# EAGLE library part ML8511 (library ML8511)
UV Sensor with Voltage Output Source: Datasheet
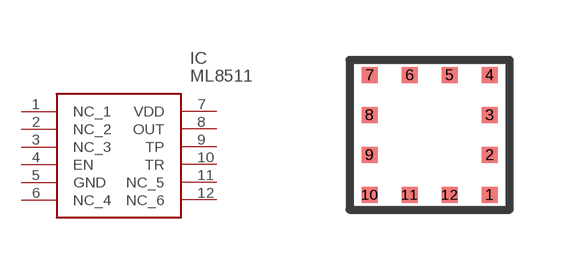
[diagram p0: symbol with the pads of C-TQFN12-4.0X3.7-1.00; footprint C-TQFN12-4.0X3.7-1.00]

Designator prefix IC

## ML8511 (Description: UV Sensor with Voltage Output; Height: mm; Manufacturer_Name: LAPIS SEMICONDUCTOR; Manufacturer_Part_Number: ML8511)  [C-TQFN12-4.0X3.7-1.00]
1  NC_1
2  NC_2
3  NC_3
4  EN
5  GND  pwr
6  NC_4
7  VDD  pwr
8  OUT  out
9  TP
10  TR
11  NC_5
12  NC_6

## Footprint C-TQFN12-4.0X3.7-1.00 (pad centres in mm)
C-TQFN12-4.0X3.7-1.00
smd 0.4 x 0.4: 1 1.5,-1.5; 2 1.5,-0.5; 3 1.5,0.5; 4 1.5,1.5; 5 0.5,1.5; 6 -0.5,1.5; 7 -1.5,1.5; 8 -1.5,0.5; 9 -1.5,-0.5; 10 -1.5,-1.5; 11 -0.5,-1.5; 12 0.5,-1.5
